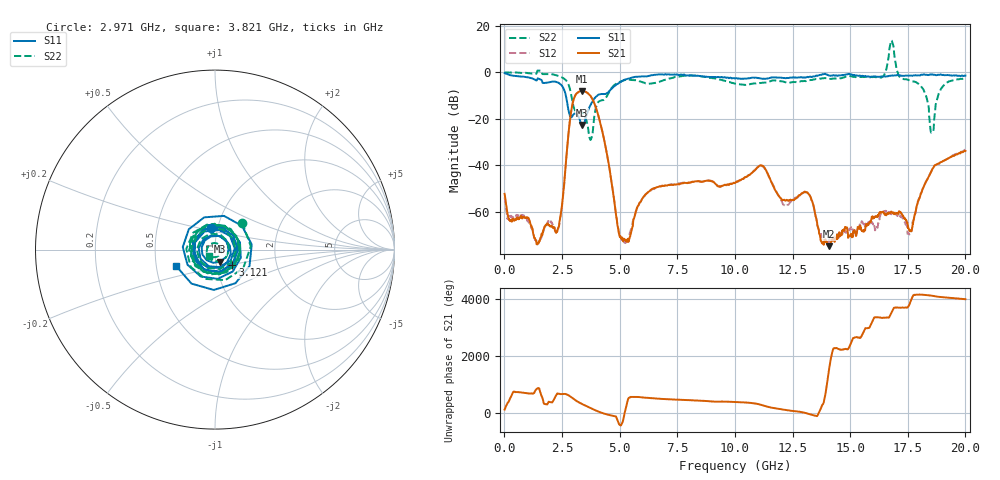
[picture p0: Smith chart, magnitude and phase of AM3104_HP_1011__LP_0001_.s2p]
!Created with skrf (http://scikit-rf.org).
# Hz S RI R 50.0
!freq ReS11 ImS11 ReS21 ImS21 ReS12 ImS12 ReS22 ImS22
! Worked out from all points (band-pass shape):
!   1601 points, 10 MHz to 20 GHz, reference 50 ohm
!   highest |S21| = -8.02 dB at 3.371 GHz (marker M1); lowest = -74.7 dB at 14.08 GHz (marker M2)
!   |S21| within 3 dB of the highest: 3.028 GHz to 3.79 GHz (761.5 MHz wide, 22.3 % of centre)
!   lowest |S11| = -22.6 dB at 3.371 GHz (marker M3), VSWR 1.16, Z = 52.5 - j7.15 ohm
!   |S11| at or under -10 dB: 2.666 GHz to 4.032 GHz (1.365 GHz wide, 40.8 % of centre)
!   |S22| runs from -29.0 to 13.7 dB; largest |S21 - S12| = 0.015
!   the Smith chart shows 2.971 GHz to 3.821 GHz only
!   S11 on the Smith chart (normalised r, x): 2.971 GHz: 0.93, +0.22; 3.121 GHz: 1.20, -0.20; 3.821 GHz: 0.63, -0.12
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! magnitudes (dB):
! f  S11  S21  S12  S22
! 10 MHz  -0.3  -52.2  -53.8  0.0
! 1.422 GHz  -3.2  -73.5  -73.5  0.4
! 2.284 GHz  -4.2  -68.4  -68.1  -1.4
! 2.971 GHz  -18.4  -12.9  -12.9  -13.4
! 3.121 GHz  -17.8  -9.2  -9.2  -17.1
! 3.346 GHz  -22.5  -8.0  -8.1  -17.1
! 3.371 GHz  -22.6  -8.0  -8.1  -17.2
! 3.821 GHz  -12.6  -11.5  -11.6  -26.5
! 5.07 GHz  -4.0  -71.4  -70.7  -3.9
! 6.682 GHz  -0.9  -49.2  -49.3  -4.2
! 10.01 GHz  -2.6  -47.5  -47.6  -4.8
! 11.15 GHz  -2.7  -40.0  -40.2  -4.6
! 12.15 GHz  -2.5  -54.9  -57.3  -4.2
! 13.34 GHz  -2.0  -55.1  -55.1  -3.3
! 14.08 GHz  -1.4  -74.7  -72.7  -2.8
! 16.35 GHz  -1.8  -60.2  -60.6  -2.3
! 16.68 GHz  -1.5  -60.8  -60.0  7.2
! 17.59 GHz  -1.4  -68.1  -69.2  -3.5
! 18.21 GHz  -0.8  -48.5  -48.7  -8.2
! 18.54 GHz  -0.9  -42.1  -42.1  -26.0
! 18.99 GHz  -1.1  -38.4  -38.5  -6.5
! 20 GHz  -1.4  -33.8  -33.2  -2.5
